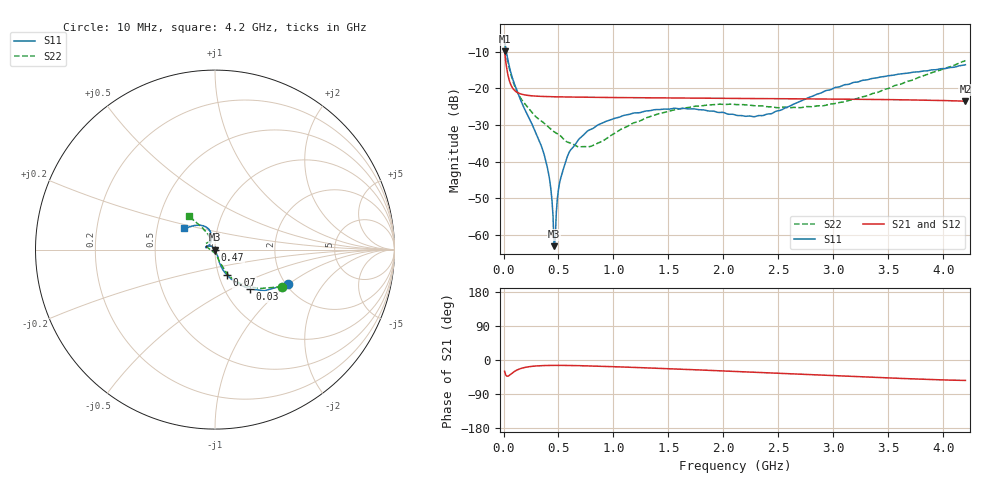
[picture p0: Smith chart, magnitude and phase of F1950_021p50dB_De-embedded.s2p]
! Integrated Device Technology
! Corporate Headquarters
! 6024 Silver Creek Valley Road
! San Jose, CA 95138  USA
! Phone:  1-408-284-8200
! Toll Free:  1-800-223-1366
! Webpage:  http://www.idt.com/
! Timing and RF Division
! 515 Groton Road, Suite 102
! Westford, MA 01886-6024
! Device:  F1950
! Description: 7-bit 0.25 dB Digital Step Attenuator
! Frequency:  150.0 -  4000.00 MHz
! Package:  4x4 mm Thin QFN Plastic Package: 24 pin
! Ports:  2 RF, 12 DC
!  Pin  1  = D0
!  Pin  2  = VDD
!  Pin  3  = Vmode
!  Pin  4  = GND
!  Pin  5  = RF1  =  Port 1
!  Pin  6  = GND
!  Pin  7  = GND
!  Pin  8  = GND
!  Pin  9  = GND
!  Pin 10  = GND
!  Pin 11  = GND
!  Pin 12  = GND
!  Pin 13  = GND
!  Pin 14  = RF2  =  Port 2
!  Pin 15  = GND
!  Pin 16  = LE
!  Pin 17  = CLK
!  Pin 18  = DATE
!  Pin 19  = D6
!  Pin 20  = D5
!  Pin 21  = D4
!  Pin 22  = D3
!  Pin 23  = D2
!  Pin 24  = D1
! State:  86
! Atten State:  21.50 dB
! Voltage:  +5.00 Volts
! Current:  Not Measured mA
! Data:  The device was measured on a the F195X evaluation board which has
!  individual transmission lines to the RF pins.  Data was collected
!  using a calibrated network analyzer.  The evaluation board was
!  de-embedded using a TRL calibration technique.
!  The reference plane is the edge of the package pin.
! Misc:  Board 2019
!  Action Tracker AT0250
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# GHz S dB R 50
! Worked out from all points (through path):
!   420 points, 10 MHz to 4.2 GHz, reference 50 ohm
!   highest |S21| = -9.87 dB at 10 MHz (marker M1); lowest = -23.5 dB at 4.2 GHz (marker M2)
!   group delay of S21, straight-line fit = 27 ps
!   lowest |S11| = -63.0 dB at 460 MHz (marker M3), VSWR 1.00, Z = 50 - j0.0683 ohm
!   |S11| at or under -10 dB: 26.17 MHz to end of sweep
!   |S22| runs from -36.0 to -7.4 dB; largest |S21 - S12| = 0.00013
!   S11 on the Smith chart (normalised r, x): 10 MHz: 2.04, -0.99; 30 MHz: 1.31, -0.63; 70 MHz: 1.09, -0.32; 470 MHz: 1.00, +0.00; 4.2 GHz: 0.69, +0.17
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0.01  -6.96 -25.5  -9.87 -30.0  -9.87 -30.0  -7.40 -29.0
0.03  -10.68 -48.5  -14.69 -42.7  -14.68 -42.7  -11.41 -49.2
0.07  -16.10 -64.8  -19.26 -36.5  -19.26 -36.6  -16.49 -63.0
0.16  -23.52 -70.9  -21.56 -22.2  -21.56 -22.2  -22.86 -69.7
0.37  -38.08 -64.3  -22.23 -14.6  -22.23 -14.6  -29.51 -75.5
0.42  -45.02 -68.8  -22.27 -14.3  -22.27 -14.3  -30.84 -77.0
0.45  -54.60 -77.6  -22.30 -14.2  -22.29 -14.2  -31.63 -80.6
0.46  -63.01 -105.0  -22.30 -14.2  -22.30 -14.2  -31.85 -82.0
0.47  -61.36 151.6  -22.31 -14.2  -22.31 -14.2  -32.02 -83.4
0.48  -53.93 135.0  -22.31 -14.2  -22.31 -14.2  -32.19 -84.4
0.51  -45.72 132.1  -22.33 -14.2  -22.33 -14.2  -32.74 -86.4
0.55  -41.43 131.0  -22.35 -14.3  -22.35 -14.3  -33.95 -89.9
0.6  -37.26 132.3  -22.37 -14.5  -22.37 -14.5  -34.84 -100.5
0.71  -33.18 135.7  -22.41 -15.1  -22.41 -15.1  -35.91 -121.7
0.81  -30.99 139.2  -22.44 -15.9  -22.45 -15.9  -35.62 -144.7
1  -28.28 146.8  -22.51 -17.7  -22.51 -17.7  -32.45 -173.9
1.41  -25.79 162.5  -22.62 -22.0  -22.61 -22.0  -26.94 163.8
2.11  -27.30 157.3  -22.75 -30.3  -22.75 -30.4  -24.43 145.3
2.43  -26.95 124.8  -22.81 -34.0  -22.81 -34.1  -25.04 134.8
2.81  -22.15 104.2  -22.89 -38.9  -22.88 -39.0  -25.01 119.3
3.51  -16.52 116.8  -23.08 -47.4  -23.07 -47.5  -19.95 115.6
4.2  -13.58 145.6  -23.50 -53.9  -23.49 -54.0  -12.46 128.3
